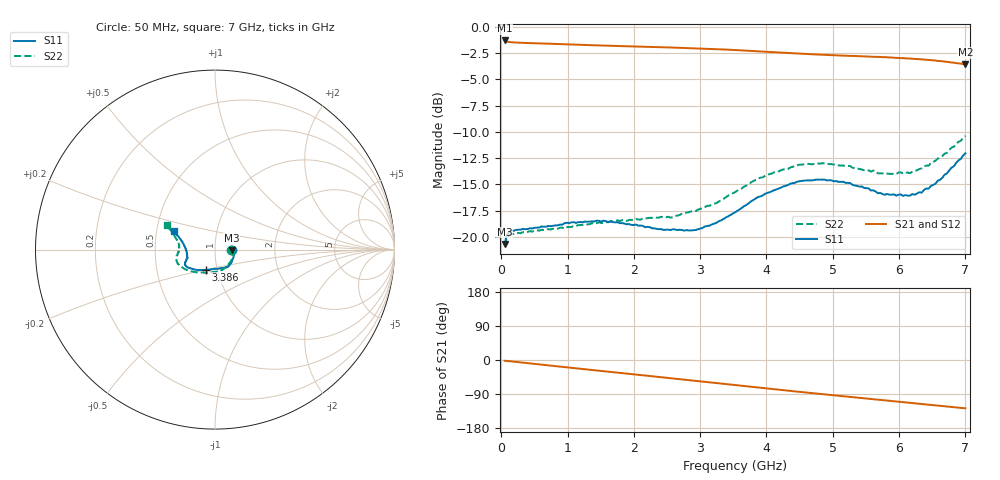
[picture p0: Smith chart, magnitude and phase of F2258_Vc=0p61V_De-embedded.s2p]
! Integrated Device Technology
! Corporate Headquarters
! 6024 Silver Creek Valley Road
! San Jose, CA 95138  USA
! Phone:  1-408-284-8200
! Toll Free:  1-800-223-1366
! Webpage:  http://www.idt.com/
! Timing and RF Division
! 515 Groton Road, Suite 102
! Westford, MA 01886-6024
! Device:  F2258
! Description: Voltage Variable RF Attenuator
! Frequency:  50.0 -  6000.00 MHz
! Package:  3x3 mm Thin QFN Plastic Package: 16 pin
! Ports:  2 RF, 2 DC
!  Pin  1  = NC
!  Pin  2  = NC
!  Pin  3  = RF2  = Port 2
!  Pin  4  = GND
!  Pin  5  = Vdd
!  Pin  6  = NC
!  Pin  7  = VCTRL
!  Pin  8  = NC
!  Pin  9  = GND
!  Pin 10  = RF1  = Port 1
!  Pin 11  = NC
!  Pin 12  = NC
!  Pin 13  = NC
!  Pin 14  = NC
!  Pin 15  = NC
!  Pin 16  = NC
! Vcntrl:  0.610 Volts
! Vdd:  +3.300 Volts
! Current:  1.107 mA
! Data:  The device was measured on a the F2258 evaluation board which has
!  individual transmission lines to the RF pins.  Data was collected
!  using a calibrated network analyzer.  The evaluation board was
!  de-embedded using a TRL calibration technique.
!  The reference plane is the edge of the package pin.
! Misc:  SN 10
!  Action Tracker AT0285
! Date Measured:  2014-12-10
! Date:  2016-01-13  MJV
! Note:
!  Integrated Device Technology supplies this data as a sample of measured
!  data at the package pin for this product.  Your particular data for this
!  product may vary.
!  Data was taken at 25 degrees C.
!  Integrated Device Technology reserves the right to change this data at anytime.
!Freq_(GHz)  S11M_(dB)  S11P_(deg)  S21M_(dB)  S21P_(deg)  S12M_(dB)  S12P_(deg)  S22M_(dB)  S22P_(deg)
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# GHz S dB R 50
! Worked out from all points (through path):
!   201 points, 50 MHz to 7 GHz, reference 50 ohm
!   highest |S21| = -1.30 dB at 50 MHz (marker M1); lowest = -3.6 dB at 7 GHz (marker M2)
!   group delay of S21, straight-line fit = 50.5 ps
!   lowest |S11| = -20.7 dB at 50 MHz (marker M3), VSWR 1.20, Z = 60.2 - j0.473 ohm
!   |S11| at or under -10 dB: start of sweep to end of sweep
!   |S22| runs from -20.9 to -10.4 dB; largest |S21 - S12| = 0.001
!   S11 on the Smith chart (normalised r, x): 50 MHz: 1.20, -0.01; 3.386 GHz: 0.88, -0.20; 7 GHz: 0.62, +0.14
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0.05  -20.67 -2.4  -1.30 -2.0  -1.30 -2.0  -20.89 -2.9
0.08475  -19.82 -4.0  -1.41 -2.5  -1.40 -2.5  -20.06 -4.5
0.15425  -19.42 -6.4  -1.47 -3.7  -1.47 -3.7  -19.72 -7.8
0.71025  -18.97 -27.3  -1.61 -14.2  -1.61 -14.2  -19.27 -32.3
1.2315  -18.62 -45.2  -1.72 -23.9  -1.72 -23.9  -18.85 -54.6
1.6485  -18.52 -55.4  -1.81 -31.5  -1.81 -31.5  -18.53 -67.5
2.37825  -19.28 -72.6  -1.94 -44.8  -1.95 -44.8  -18.17 -86.7
2.552  -19.36 -77.8  -1.98 -48.0  -1.98 -48.0  -18.18 -92.0
2.93425  -19.35 -93.2  -2.05 -55.1  -2.06 -55.1  -17.54 -105.7
3.386  -18.16 -114.1  -2.17 -63.6  -2.17 -63.6  -16.24 -124.2
3.525  -17.67 -119.8  -2.22 -66.3  -2.22 -66.3  -15.75 -129.3
4.0115  -15.82 -137.4  -2.39 -75.3  -2.39 -75.3  -14.08 -145.8
4.46325  -14.76 -147.6  -2.55 -83.5  -2.56 -83.5  -13.19 -157.6
4.7065  -14.62 -151.0  -2.63 -87.7  -2.63 -87.7  -13.08 -162.1
5.2625  -14.88 -157.4  -2.78 -97.4  -2.79 -97.4  -13.27 -170.8
5.64475  -15.68 -163.0  -2.87 -104.0  -2.87 -104.0  -13.74 -176.5
5.6795  -15.86 -162.8  -2.86 -104.6  -2.87 -104.6  -13.96 -176.8
5.85325  -16.00 -166.8  -2.92 -107.7  -2.93 -107.7  -14.00 178.5
6.166  -16.08 -175.1  -3.03 -113.3  -3.03 -113.3  -13.94 172.1
6.33975  -15.80 177.6  -3.10 -116.4  -3.11 -116.4  -13.49 167.6
6.6525  -14.38 165.8  -3.28 -121.9  -3.29 -121.9  -12.31 160.5
7  -12.05 155.5  -3.58 -127.4  -3.59 -127.4  -10.40 152.9
